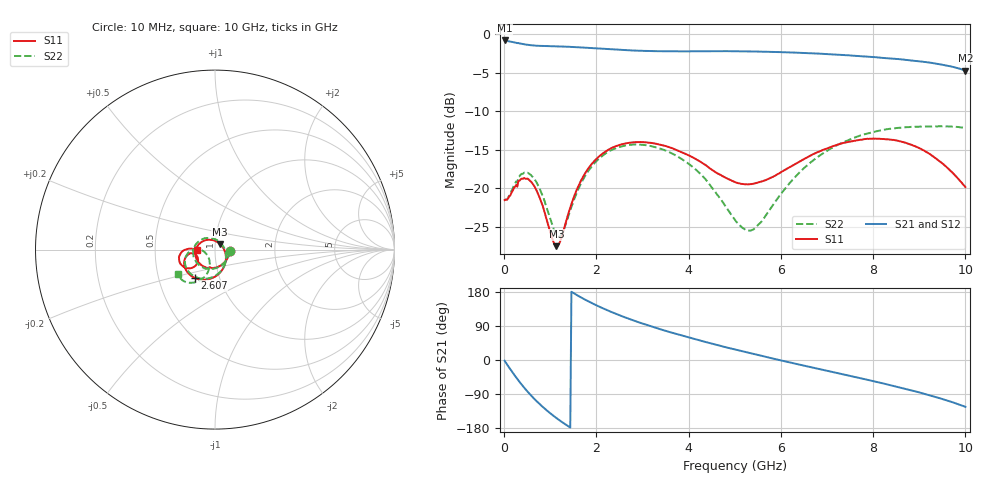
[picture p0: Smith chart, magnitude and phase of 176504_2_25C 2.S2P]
!  2-Port S-parameters saved by WinCal
! VAR MeasName=S-Parameters (CALIBRATED_DATA) read from VNA (N5242A)
! VAR MeasDate=2017-11-2 16:05:30
! VAR NAME=176504_2_25C 2
! VAR FILENAME=176504_2_25C 2.S2P
! VAR DATE=2017-11-2 16:05:30
! VAR PHYS_PORTS=2,3
# Hz S DB R 50
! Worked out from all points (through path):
!   401 points, 10 MHz to 10 GHz, reference 50 ohm
!   highest |S21| = -0.84 dB at 10 MHz (marker M1); lowest = -4.7 dB at 10 GHz (marker M2)
!   lowest |S11| = -27.6 dB at 1.134 GHz (marker M3), VSWR 1.09, Z = 52.7 + j3.35 ohm
!   |S11| at or under -10 dB: start of sweep to end of sweep
!   |S22| runs from -26.3 to -12.0 dB; largest |S21 - S12| = 0.0076
!   S11 on the Smith chart (normalised r, x): 10 MHz: 1.18, -0.02; 2.607 GHz: 0.76, -0.25; 10 GHz: 0.82, -0.00
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1e7  -21.56 -4.6  -0.84 -2.0  -0.84 -2.0  -21.54 -4.6
1.34875e8  -20.95 -59.0  -0.99 -24.6  -0.99 -24.6  -20.76 -61.5
2.5975e8  -19.61 -100.0  -1.14 -45.9  -1.14 -45.9  -19.14 -102.6
3.5965e8  -18.86 -125.7  -1.24 -61.8  -1.25 -61.9  -18.26 -128.3
4.84525e8  -18.80 -153.9  -1.39 -80.2  -1.39 -80.2  -18.05 -156.1
6.34375e8  -19.59 177.1  -1.49 -100.1  -1.49 -100.1  -18.67 175.2
8.092e8  -21.91 143.6  -1.55 -120.7  -1.55 -120.7  -20.65 142.5
1.133875e9  -27.55 49.1  -1.60 -153.3  -1.59 -153.2  -26.11 59.1
1.25875e9  -26.14 3.7  -1.62 -164.1  -1.62 -164.1  -25.87 15.0
1.683325e9  -18.85 -66.8  -1.75 164.0  -1.75 164.0  -19.21 -64.4
2.132875e9  -15.53 -101.1  -1.93 136.8  -1.93 136.8  -15.80 -101.4
2.6074e9  -14.24 -125.9  -2.09 113.1  -2.09 113.1  -14.51 -127.8
3.35665e9  -14.34 -152.9  -2.23 82.2  -2.25 82.2  -14.83 -157.5
4.2058e9  -16.40 -169.8  -2.23 52.7  -2.24 52.8  -17.89 -179.0
5.005e9  -19.23 -163.9  -2.24 27.6  -2.23 27.7  -24.14 -169.8
5.429575e9  -19.40 -152.6  -2.27 15.1  -2.27 15.2  -25.25 -134.2
6.05395e9  -17.77 -141.5  -2.36 -2.6  -2.37 -2.5  -20.36 -107.9
6.678325e9  -15.66 -141.7  -2.51 -19.7  -2.52 -19.7  -16.50 -109.1
7.577425e9  -13.89 -152.8  -2.82 -44.1  -2.85 -44.0  -13.50 -120.9
8.35165e9  -13.70 -166.2  -3.16 -65.6  -3.22 -65.6  -12.32 -131.4
9.25075e9  -15.68 180.0  -3.74 -93.9  -3.75 -93.6  -12.02 -140.1
1e10  -19.88 -178.7  -4.74 -123.5  -4.76 -123.2  -12.19 -146.3
